FUNCTION_BLOCK "IMAC_MOTOR2_CALL"
TITLE =Function calls for MOTOR2 objects
//Parameter Description for Function MOTOR2 (FB81):
//-------------------------------------------------
//OBJ:     Ascending Object number for MOTOR2 (1...x)
//
//RMOT:    'REMOTE'     Feedback
//                      0 = Local
//                      1 = Remote)
//
//RUN1:     'RUN'       Feedback 'Low Speed' or 'Forward'
//                      0 = Stopped
//                      1 = Running in 'Low Speed' or 'Forward Direction'
//
//RUN2:     'RUN'       Feedback 'High Speed' or Reverse'
//                      0 = Stopped
//                      1 = Running in 'High Speed' or 'Reverse Direction'
//
//FAUL:     'EXT.FAULT' Feedback
//                      0 = OK
//                      1 = Fault
//
//ACOM:    'AUTO' Mode  Command Interface (only active, if 'REMOTE'+'AUTO')
//                      Bit  0       : BlackoutStart Command
//                      Bit  7       : FetchData Command (from Standby Unit)
//                      Bit  8       : Start1 Command ('Low Speed' or 'Forward')
//                      Bit  9       : Stop Command
//                      Bit 10       : Failure input from Automatic Function
//                      Bit 11       : Lock Start/Stop Commands
//                      Bit 12       : Emergency Off
//                      Bit 13       : Start2 Command ('High Speed' or 'Reverse')
//
//BLKO:    'BLACKOUT'   Feedback
//                      0 = No Blackout
//                      1 = Blackout
//
//PCONF:   (leave empty, refers to local instance data in Instance DB)
//
//MST1:    'START1'     Output to Motor for 'Low Speed' or 'Forward'
//                      0 = No Command
//                      1 = Start1 Command
//
//MST2:    'START2'     Output to Motor for 'High Speed' or 'Reverse'
//                      0 = No Command
//                      1 = Start2 Command
//
//MSTO:    'STOP'       Output to Motor
//                      0 = No Command
//                      1 = Stop Command
//
//STAT:   'AUTO' Mode  Status Interface
//                      Bit  0       : Running 2  ('High Speed' or 'Reverse')
//                      Bit  1       : Starting 2 ('High Speed' or 'Reverse')
//                      Bit  8       : Running 1  ('Low Speed' or 'Forward')
//                      Bit  9       : Local
//                      Bit 10       : Manual
//                      Bit 11       : Auto
//                      Bit 12       : Failure
//                      Bit 13       : BlackOut
//                      Bit 14       : Starting1  ('Low Speed' or 'Forward')
//                      Bit 15       : Restarting
//
//OSSTAT:  OS Status Word
//                      Value = 0    : Undefined
//                      Value = 1    : Running1    ('Low Speed' or 'Forward')
//                      Value = 2    : Running2    ('High Speed' or 'Reverse')
//                      Value = 3    : Stopped
//                      Value = 4    : Starting1   ('Low Speed' or 'Forward')
//                      Value = 5    : Starting2   ('High Speed' or 'Reverse')
//                      Value = 7    : Blackout
//                      Value + 256  : Local Mode  (Offset Value)
//                      Value + 512  : Manual Mode (Offset Value)
//                      Value + 1024 : Auto Mode   (Offset Value)
//
//OSALARM: OS Alarm Word
//                      Value = 0    : Undefined
//                      Value = 1    : Normal
//                      Value = 2    : External Fault Alarm
//                      Value = 3    : Auto Failure Alarm
//                      Value = 4    : Action Alarm
//                      Value = 5    : Non-Feedback Alarm
//                      Value = 6    : Lock
//                      Value = 7    : Emergency Off
//                      Value = 8    : Blackout
//
//OSCOM:   OS Command Interface
//                      Bit  0       : Start1 Command ('Low Speed' or 'Forward')
//                      Bit  1       : Start2 Command ('High Speed' or 'Reverse')
//                      Bit  2       : Stop   Command from OS
//                      Bit  7       : Reset  Command from OS
//                      Bit  9       : Manual Command from OS
//                      Bit 10       : Auto   Command from OS
AUTHOR : Kahle
FAMILY : IMAC
VERSION : 0.1


VAR
  MotorNo_001 : "IMAC_MOTOR2";
  MotorNo_002 : "IMAC_MOTOR2";
  MotorNo_003 : "IMAC_MOTOR2";
  MotorNo_004 : "IMAC_MOTOR2";
  MotorNo_005 : "IMAC_MOTOR2";
  MotorNo_006 : "IMAC_MOTOR2";
  MotorNo_007 : "IMAC_MOTOR2";
  MotorNo_008 : "IMAC_MOTOR2";
  MotorNo_009 : "IMAC_MOTOR2";
  MotorNo_010 : "IMAC_MOTOR2";
  MotorNo_011 : "IMAC_MOTOR2";
  MotorNo_012 : "IMAC_MOTOR2";
  MotorNo_013 : "IMAC_MOTOR2";
  MotorNo_014 : "IMAC_MOTOR2";
  MotorNo_015 : "IMAC_MOTOR2";
  MotorNo_016 : "IMAC_MOTOR2";
  MotorNo_017 : "IMAC_MOTOR2";
  MotorNo_018 : "IMAC_MOTOR2";
  MotorNo_019 : "IMAC_MOTOR2";
  MotorNo_020 : "IMAC_MOTOR2";
  MotorNo_021 : "IMAC_MOTOR2";
  MotorNo_022 : "IMAC_MOTOR2";
  MotorNo_023 : "IMAC_MOTOR2";
  MotorNo_024 : "IMAC_MOTOR2";
  MotorNo_025 : "IMAC_MOTOR2";
END_VAR
BEGIN
NETWORK
TITLE =MOTOR2 Number 001

      CALL #MotorNo_001 (
           OBJ                      := 1,
           RMOT                     := E      5.0,
           RUN1                     := E      5.1,
           RUN2                     := E      5.2,
           FAUL                     := E      5.3,
           ACOM                     := "IMAC_MOTOR2_I/O".MOTOR2_001_ACOM,
           BLKO                     := E      5.4,
           MST1                     := A      2.0,
           MST2                     := A      2.1,
           MSTO                     := A      2.2,
           STAT                     := "IMAC_MOTOR2_I/O".MOTOR2_001_STAT,
           OSSTAT                   := "IMAC_MOTOR2_I/O".MOTOR2_001_OSSTAT,
           OSALARM                  := "IMAC_MOTOR2_I/O".MOTOR2_001_OSALARM,
           OSCOM                    := "IMAC_MOTOR2_I/O".MOTOR2_001_OSCOM);

NETWORK
TITLE =MOTOR2 Number 002

      CALL #MotorNo_002 (
           OBJ                      := 2,
           RMOT                     := E      5.5,
           RUN1                     := E      5.6,
           RUN2                     := E      5.7,
           FAUL                     := E      6.0,
           ACOM                     := "IMAC_MOTOR2_I/O".MOTOR2_002_ACOM,
           BLKO                     := E      6.1,
           MST1                     := A      2.3,
           MST2                     := A      2.4,
           MSTO                     := A      2.5,
           STAT                     := "IMAC_MOTOR2_I/O".MOTOR2_002_STAT,
           OSSTAT                   := "IMAC_MOTOR2_I/O".MOTOR2_002_OSSTAT,
           OSALARM                  := "IMAC_MOTOR2_I/O".MOTOR2_002_OSALARM,
           OSCOM                    := "IMAC_MOTOR2_I/O".MOTOR2_002_OSCOM);

NETWORK
TITLE =MOTOR2 Number 003

      CALL #MotorNo_003 (
           OBJ                      := 3,
           RMOT                     := E      6.2,
           RUN1                     := E      6.3,
           RUN2                     := E      6.4,
           FAUL                     := E      6.5,
           ACOM                     := "IMAC_MOTOR2_I/O".MOTOR2_003_ACOM,
           BLKO                     := E      6.6,
           MST1                     := A      2.6,
           MST2                     := A      2.7,
           MSTO                     := A      3.0,
           STAT                     := "IMAC_MOTOR2_I/O".MOTOR2_003_STAT,
           OSSTAT                   := "IMAC_MOTOR2_I/O".MOTOR2_003_OSSTAT,
           OSALARM                  := "IMAC_MOTOR2_I/O".MOTOR2_003_OSALARM,
           OSCOM                    := "IMAC_MOTOR2_I/O".MOTOR2_003_OSCOM);

NETWORK
TITLE =MOTOR2 Number 004

//*********** END of Function Processing ! *******************************************************************
      BEA   ; // Move this Instruction down to the next Network to add one object !
//************************************************************************************************************

      CALL #MotorNo_004 (
           OBJ                      := 4,
           ACOM                     := "IMAC_MOTOR2_I/O".MOTOR2_004_ACOM,
           STAT                     := "IMAC_MOTOR2_I/O".MOTOR2_004_STAT,
           OSSTAT                   := "IMAC_MOTOR2_I/O".MOTOR2_004_OSSTAT,
           OSALARM                  := "IMAC_MOTOR2_I/O".MOTOR2_004_OSALARM,
           OSCOM                    := "IMAC_MOTOR2_I/O".MOTOR2_004_OSCOM);

NETWORK
TITLE =MOTOR2 Number 005

      CALL #MotorNo_005 (
           OBJ                      := 5,
           ACOM                     := "IMAC_MOTOR2_I/O".MOTOR2_005_ACOM,
           STAT                     := "IMAC_MOTOR2_I/O".MOTOR2_005_STAT,
           OSSTAT                   := "IMAC_MOTOR2_I/O".MOTOR2_005_OSSTAT,
           OSALARM                  := "IMAC_MOTOR2_I/O".MOTOR2_005_OSALARM,
           OSCOM                    := "IMAC_MOTOR2_I/O".MOTOR2_005_OSCOM);

NETWORK
TITLE =MOTOR2 Number 006

      CALL #MotorNo_006 (
           OBJ                      := 6,
           ACOM                     := "IMAC_MOTOR2_I/O".MOTOR2_006_ACOM,
           STAT                     := "IMAC_MOTOR2_I/O".MOTOR2_006_STAT,
           OSSTAT                   := "IMAC_MOTOR2_I/O".MOTOR2_006_OSSTAT,
           OSALARM                  := "IMAC_MOTOR2_I/O".MOTOR2_006_OSALARM,
           OSCOM                    := "IMAC_MOTOR2_I/O".MOTOR2_006_OSCOM);

NETWORK
TITLE =MOTOR2 Number 007

      CALL #MotorNo_007 (
           OBJ                      := 7,
           ACOM                     := "IMAC_MOTOR2_I/O".MOTOR2_007_ACOM,
           STAT                     := "IMAC_MOTOR2_I/O".MOTOR2_007_STAT,
           OSSTAT                   := "IMAC_MOTOR2_I/O".MOTOR2_007_OSSTAT,
           OSALARM                  := "IMAC_MOTOR2_I/O".MOTOR2_007_OSALARM,
           OSCOM                    := "IMAC_MOTOR2_I/O".MOTOR2_007_OSCOM);

NETWORK
TITLE =MOTOR2 Number 008

      CALL #MotorNo_008 (
           OBJ                      := 8,
           ACOM                     := "IMAC_MOTOR2_I/O".MOTOR2_008_ACOM,
           STAT                     := "IMAC_MOTOR2_I/O".MOTOR2_008_STAT,
           OSSTAT                   := "IMAC_MOTOR2_I/O".MOTOR2_008_OSSTAT,
           OSALARM                  := "IMAC_MOTOR2_I/O".MOTOR2_008_OSALARM,
           OSCOM                    := "IMAC_MOTOR2_I/O".MOTOR2_008_OSCOM);

NETWORK
TITLE =MOTOR2 Number 009

      CALL #MotorNo_009 (
           OBJ                      := 9,
           ACOM                     := "IMAC_MOTOR2_I/O".MOTOR2_009_ACOM,
           STAT                     := "IMAC_MOTOR2_I/O".MOTOR2_009_STAT,
           OSSTAT                   := "IMAC_MOTOR2_I/O".MOTOR2_009_OSSTAT,
           OSALARM                  := "IMAC_MOTOR2_I/O".MOTOR2_009_OSALARM,
           OSCOM                    := "IMAC_MOTOR2_I/O".MOTOR2_009_OSCOM);

NETWORK
TITLE =MOTOR2 Number 010

      CALL #MotorNo_010 (
           OBJ                      := 10,
           ACOM                     := "IMAC_MOTOR2_I/O".MOTOR2_010_ACOM,
           STAT                     := "IMAC_MOTOR2_I/O".MOTOR2_010_STAT,
           OSSTAT                   := "IMAC_MOTOR2_I/O".MOTOR2_010_OSSTAT,
           OSALARM                  := "IMAC_MOTOR2_I/O".MOTOR2_010_OSALARM,
           OSCOM                    := "IMAC_MOTOR2_I/O".MOTOR2_010_OSCOM);

NETWORK
TITLE =MOTOR2 Number 011

      CALL #MotorNo_011 (
           OBJ                      := 11,
           ACOM                     := "IMAC_MOTOR2_I/O".MOTOR2_011_ACOM,
           STAT                     := "IMAC_MOTOR2_I/O".MOTOR2_011_STAT,
           OSSTAT                   := "IMAC_MOTOR2_I/O".MOTOR2_011_OSSTAT,
           OSALARM                  := "IMAC_MOTOR2_I/O".MOTOR2_011_OSALARM,
           OSCOM                    := "IMAC_MOTOR2_I/O".MOTOR2_011_OSCOM);

NETWORK
TITLE =MOTOR2 Number 012

      CALL #MotorNo_012 (
           OBJ                      := 12,
           ACOM                     := "IMAC_MOTOR2_I/O".MOTOR2_012_ACOM,
           STAT                     := "IMAC_MOTOR2_I/O".MOTOR2_012_STAT,
           OSSTAT                   := "IMAC_MOTOR2_I/O".MOTOR2_012_OSSTAT,
           OSALARM                  := "IMAC_MOTOR2_I/O".MOTOR2_012_OSALARM,
           OSCOM                    := "IMAC_MOTOR2_I/O".MOTOR2_012_OSCOM);

NETWORK
TITLE =MOTOR2 Number 013

      CALL #MotorNo_013 (
           OBJ                      := 13,
           ACOM                     := "IMAC_MOTOR2_I/O".MOTOR2_013_ACOM,
           STAT                     := "IMAC_MOTOR2_I/O".MOTOR2_013_STAT,
           OSSTAT                   := "IMAC_MOTOR2_I/O".MOTOR2_013_OSSTAT,
           OSALARM                  := "IMAC_MOTOR2_I/O".MOTOR2_013_OSALARM,
           OSCOM                    := "IMAC_MOTOR2_I/O".MOTOR2_013_OSCOM);

NETWORK
TITLE =MOTOR2 Number 014

      CALL #MotorNo_014 (
           OBJ                      := 14,
           ACOM                     := "IMAC_MOTOR2_I/O".MOTOR2_014_ACOM,
           STAT                     := "IMAC_MOTOR2_I/O".MOTOR2_014_STAT,
           OSSTAT                   := "IMAC_MOTOR2_I/O".MOTOR2_014_OSSTAT,
           OSALARM                  := "IMAC_MOTOR2_I/O".MOTOR2_014_OSALARM,
           OSCOM                    := "IMAC_MOTOR2_I/O".MOTOR2_014_OSCOM);

NETWORK
TITLE =MOTOR2 Number 015

      CALL #MotorNo_015 (
           OBJ                      := 15,
           ACOM                     := "IMAC_MOTOR2_I/O".MOTOR2_015_ACOM,
           STAT                     := "IMAC_MOTOR2_I/O".MOTOR2_015_STAT,
           OSSTAT                   := "IMAC_MOTOR2_I/O".MOTOR2_015_OSSTAT,
           OSALARM                  := "IMAC_MOTOR2_I/O".MOTOR2_015_OSALARM,
           OSCOM                    := "IMAC_MOTOR2_I/O".MOTOR2_015_OSCOM);

NETWORK
TITLE =MOTOR2 Number 016

      CALL #MotorNo_016 (
           OBJ                      := 16,
           ACOM                     := "IMAC_MOTOR2_I/O".MOTOR2_016_ACOM,
           STAT                     := "IMAC_MOTOR2_I/O".MOTOR2_016_STAT,
           OSSTAT                   := "IMAC_MOTOR2_I/O".MOTOR2_016_OSSTAT,
           OSALARM                  := "IMAC_MOTOR2_I/O".MOTOR2_016_OSALARM,
           OSCOM                    := "IMAC_MOTOR2_I/O".MOTOR2_016_OSCOM);

NETWORK
TITLE =MOTOR2 Number 017

      CALL #MotorNo_017 (
           OBJ                      := 17,
           ACOM                     := "IMAC_MOTOR2_I/O".MOTOR2_017_ACOM,
           STAT                     := "IMAC_MOTOR2_I/O".MOTOR2_017_STAT,
           OSSTAT                   := "IMAC_MOTOR2_I/O".MOTOR2_017_OSSTAT,
           OSALARM                  := "IMAC_MOTOR2_I/O".MOTOR2_017_OSALARM,
           OSCOM                    := "IMAC_MOTOR2_I/O".MOTOR2_017_OSCOM);

NETWORK
TITLE =MOTOR2 Number 018

      CALL #MotorNo_018 (
           OBJ                      := 18,
           ACOM                     := "IMAC_MOTOR2_I/O".MOTOR2_018_ACOM,
           STAT                     := "IMAC_MOTOR2_I/O".MOTOR2_018_STAT,
           OSSTAT                   := "IMAC_MOTOR2_I/O".MOTOR2_018_OSSTAT,
           OSALARM                  := "IMAC_MOTOR2_I/O".MOTOR2_018_OSALARM,
           OSCOM                    := "IMAC_MOTOR2_I/O".MOTOR2_018_OSCOM);

NETWORK
TITLE =MOTOR2 Number 019

      CALL #MotorNo_019 (
           OBJ                      := 19,
           ACOM                     := "IMAC_MOTOR2_I/O".MOTOR2_019_ACOM,
           STAT                     := "IMAC_MOTOR2_I/O".MOTOR2_019_STAT,
           OSSTAT                   := "IMAC_MOTOR2_I/O".MOTOR2_019_OSSTAT,
           OSALARM                  := "IMAC_MOTOR2_I/O".MOTOR2_019_OSALARM,
           OSCOM                    := "IMAC_MOTOR2_I/O".MOTOR2_019_OSCOM);

NETWORK
TITLE =MOTOR2 Number 020

      CALL #MotorNo_020 (
           OBJ                      := 20,
           ACOM                     := "IMAC_MOTOR2_I/O".MOTOR2_020_ACOM,
           STAT                     := "IMAC_MOTOR2_I/O".MOTOR2_020_STAT,
           OSSTAT                   := "IMAC_MOTOR2_I/O".MOTOR2_020_OSSTAT,
           OSALARM                  := "IMAC_MOTOR2_I/O".MOTOR2_020_OSALARM,
           OSCOM                    := "IMAC_MOTOR2_I/O".MOTOR2_020_OSCOM);

NETWORK
TITLE =MOTOR2 Number 021

      CALL #MotorNo_021 (
           OBJ                      := 21,
           ACOM                     := "IMAC_MOTOR2_I/O".MOTOR2_021_ACOM,
           STAT                     := "IMAC_MOTOR2_I/O".MOTOR2_021_STAT,
           OSSTAT                   := "IMAC_MOTOR2_I/O".MOTOR2_021_OSSTAT,
           OSALARM                  := "IMAC_MOTOR2_I/O".MOTOR2_021_OSALARM,
           OSCOM                    := "IMAC_MOTOR2_I/O".MOTOR2_021_OSCOM);

NETWORK
TITLE =MOTOR2 Number 022

      CALL #MotorNo_022 (
           OBJ                      := 22,
           ACOM                     := "IMAC_MOTOR2_I/O".MOTOR2_022_ACOM,
           STAT                     := "IMAC_MOTOR2_I/O".MOTOR2_022_STAT,
           OSSTAT                   := "IMAC_MOTOR2_I/O".MOTOR2_022_OSSTAT,
           OSALARM                  := "IMAC_MOTOR2_I/O".MOTOR2_022_OSALARM,
           OSCOM                    := "IMAC_MOTOR2_I/O".MOTOR2_022_OSCOM);

NETWORK
TITLE =MOTOR2 Number 023

      CALL #MotorNo_023 (
           OBJ                      := 23,
           ACOM                     := "IMAC_MOTOR2_I/O".MOTOR2_023_ACOM,
           STAT                     := "IMAC_MOTOR2_I/O".MOTOR2_023_STAT,
           OSSTAT                   := "IMAC_MOTOR2_I/O".MOTOR2_023_OSSTAT,
           OSALARM                  := "IMAC_MOTOR2_I/O".MOTOR2_023_OSALARM,
           OSCOM                    := "IMAC_MOTOR2_I/O".MOTOR2_023_OSCOM);

NETWORK
TITLE =MOTOR2 Number 024

      CALL #MotorNo_024 (
           OBJ                      := 24,
           ACOM                     := "IMAC_MOTOR2_I/O".MOTOR2_024_ACOM,
           STAT                     := "IMAC_MOTOR2_I/O".MOTOR2_024_STAT,
           OSSTAT                   := "IMAC_MOTOR2_I/O".MOTOR2_024_OSSTAT,
           OSALARM                  := "IMAC_MOTOR2_I/O".MOTOR2_024_OSALARM,
           OSCOM                    := "IMAC_MOTOR2_I/O".MOTOR2_024_OSCOM);

NETWORK
TITLE =MOTOR2 Number 025

      CALL #MotorNo_025 (
           OBJ                      := 25,
           ACOM                     := "IMAC_MOTOR2_I/O".MOTOR2_025_ACOM,
           STAT                     := "IMAC_MOTOR2_I/O".MOTOR2_025_STAT,
           OSSTAT                   := "IMAC_MOTOR2_I/O".MOTOR2_025_OSSTAT,
           OSALARM                  := "IMAC_MOTOR2_I/O".MOTOR2_025_OSALARM,
           OSCOM                    := "IMAC_MOTOR2_I/O".MOTOR2_025_OSCOM);

END_FUNCTION_BLOCK

